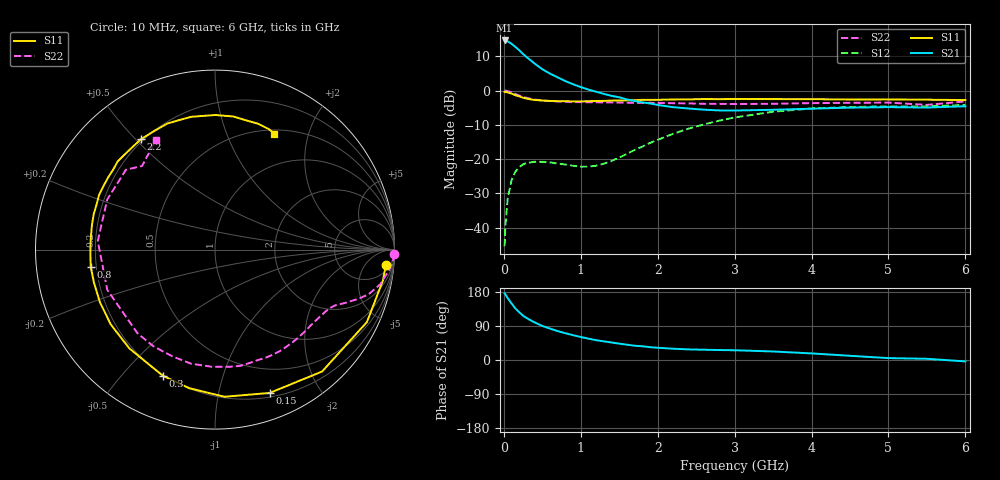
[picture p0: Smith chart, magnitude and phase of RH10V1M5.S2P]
! SIEMENS Small Signal Semiconductors
! BFR106
! Si NPN RF Bipolar Junction Transistor in SOT23
! VCE = 10 V  IC = 1.5 mA
! Common Emitter S-Parameters:  August  1996
# GHz  S  MA  R  50
!  f  S11  S21  S12  S22
! GHz  MAG  ANG  MAG  ANG  MAG  ANG  MAG  ANG
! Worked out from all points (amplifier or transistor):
!   36 points, 10 MHz to 6 GHz, reference 50 ohm
!   highest |S21| = 14.6 dB at 10 MHz (marker M1)
!   |S21| within 3 dB of that: start of sweep to 206.2 MHz
!   unconditionally stable (mu >= 1): 826.5 MHz to 1.807 GHz; 3.884 GHz to end of sweep
!   at 250 MHz: K = 0.29, MSG = 16.1 dB, |S12| = -21.5 dB
!   at 1.4 GHz: K = 1.28, MAG = 6.3 dB, |S12| = -20.5 dB
!   at 6 GHz: K = 1.02, MAG = -1.1 dB, |S12| = -4.2 dB
!   S11 on the Smith chart (normalised r, x): 10 MHz: 9, -17; 150 MHz: 0.24, -1.42; 300 MHz: 0.20, -0.65; 800 MHz: 0.18, -0.07; 2.2 GHz: 0.19, +0.52; 6 GHz: 0.55, +1.49
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0.01  0.9549 -5.3  5.363 175.9  0.0054 89.8  0.9991 -1.5
0.02  0.9518 -10.3  5.362 173.5  0.0106 83.2  0.9976 -2.7
0.05  0.9378 -25.5  5.191 163.2  0.0266 76.4  0.9794 -6.4
0.1  0.9041 -48.7  4.795 149.4  0.0493 64.1  0.9403 -11.9
0.15  0.8548 -69.1  4.331 135.8  0.0659 53.0  0.8916 -16.2
0.2  0.8216 -86.3  3.855 126.1  0.0764 45.6  0.8468 -18.8
0.25  0.7853 -100.5  3.408 116.9  0.084 39.1  0.8076 -20.9
0.3  0.7604 -112.5  3.04 110.2  0.0883 35.2  0.7795 -22.5
0.4  0.7285 -130.9  2.471 99.2  0.0916 28.7  0.738 -24.9
0.5  0.715 -144.3  2.044 90.0  0.0914 25.5  0.7151 -27.3
0.6  0.7051 -155.4  1.763 82.7  0.0898 24.3  0.7028 -30.0
0.8  0.699 -172.2  1.372 70.6  0.0835 27.3  0.6853 -35.8
1.1  0.6992 168.7  1.032 56.4  0.0779 43.1  0.6752 -45.8
1.6  0.7185 145.9  0.742 40.4  0.1197 73.0  0.6652 -64.8
2.2  0.7409 123.7  0.572 29.8  0.2341 75.3  0.6532 -91.5
2.8  0.7486 105.3  0.513 26.3  0.3636 63.1  0.6388 -122.6
3.5  0.7499 89.9  0.524 22.5  0.4914 45.2  0.6408 -159.5
4  0.7486 82.2  0.544 17.4  0.5474 32.6  0.6549 175.8
4.5  0.7404 76.1  0.563 11.1  0.575 21.5  0.6622 155.1
5  0.7414 71.1  0.573 5.0  0.5878 12.3  0.6666 138.1
5.5  0.7353 66.0  0.565 3.2  0.5861 7.9  0.6181 131.1
6  0.7259 62.9  0.59 -3.7  0.6173 -0.4  0.6938 118.4
